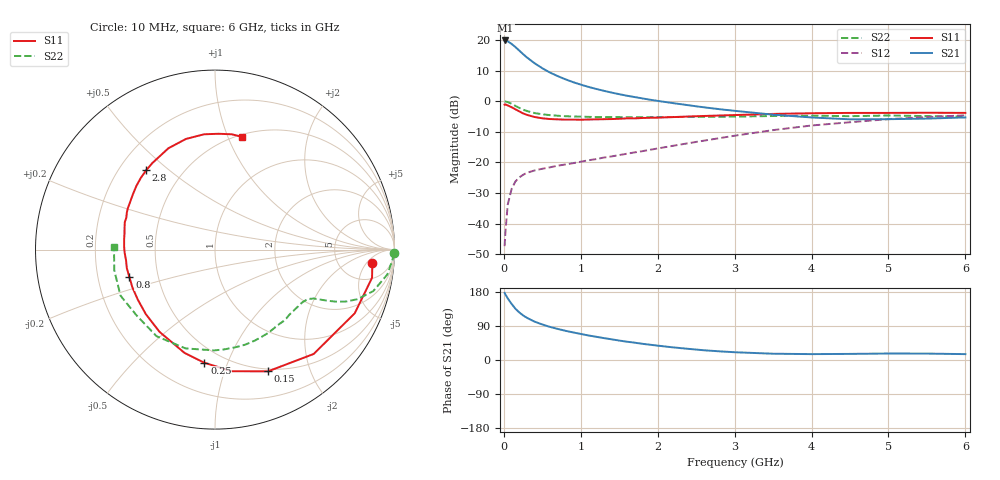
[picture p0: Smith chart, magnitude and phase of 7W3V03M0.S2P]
! Infineon Technologies  Discrete & RF Semiconductors
! BFS17W
! Si NPN RF Bipolar Junction Transistor in SOT323
! VCE = 3 V  IC = 3 mA
! Common Emitter S-Parameters:  August  1999
# GHz  S  MA  R  50
!  f  S11  S21  S12  S22
! GHz  MAG  ANG  MAG  ANG  MAG  ANG  MAG  ANG
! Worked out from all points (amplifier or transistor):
!   36 points, 10 MHz to 6 GHz, reference 50 ohm
!   highest |S21| = 19.9 dB at 20 MHz (marker M1)
!   |S21| within 3 dB of that: start of sweep to 187.2 MHz
!   unconditionally stable (mu >= 1): 699.9 MHz to 3.232 GHz; 4.015 GHz to end of sweep
!   at 250 MHz: K = 0.45, MSG = 19.7 dB, |S12| = -24.0 dB
!   at 1.4 GHz: K = 1.29, MAG = 7.2 dB, |S12| = -18.0 dB
!   at 6 GHz: K = 1.09, MAG = -2.2 dB, |S12| = -4.6 dB
!   S11 on the Smith chart (normalised r, x): 10 MHz: 11, -7; 150 MHz: 0.47, -1.42; 250 MHz: 0.39, -0.83; 800 MHz: 0.34, -0.14; 2.8 GHz: 0.31, +0.42; 6 GHz: 0.52, +1.12
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0.01  0.8798 -4.9  9.833 177.1  0.0043 85.5  0.9971 -1.2
0.02  0.889 -10.2  9.842 173.1  0.0071 85.8  0.9899 -3.4
0.05  0.8555 -24.5  9.54 162.9  0.0203 77.7  0.9704 -8.2
0.1  0.8003 -46.6  8.658 148.2  0.0367 65.7  0.9116 -14.7
0.15  0.7397 -66.5  7.69 135.4  0.0489 57.6  0.8405 -19.2
0.2  0.6843 -82.0  6.736 125.7  0.057 52.4  0.781 -21.8
0.25  0.6336 -95.3  5.896 117.7  0.0629 48.0  0.7293 -23.4
0.3  0.6002 -106.4  5.2 111.4  0.0678 45.8  0.6939 -24.3
0.4  0.5527 -124.0  4.176 101.2  0.0742 43.4  0.6419 -25.6
0.5  0.5271 -137.0  3.461 93.7  0.079 42.9  0.6125 -26.4
0.6  0.5125 -147.0  2.943 87.3  0.0834 43.8  0.5931 -27.6
0.8  0.5011 -162.1  2.285 77.1  0.0928 46.7  0.57 -30.8
0.9  0.502 -168.1  2.053 72.8  0.0975 48.2  0.5637 -32.6
1.1  0.5038 -178.1  1.717 64.7  0.1087 51.2  0.5562 -36.8
1.3  0.5097 173.3  1.483 57.8  0.1204 53.8  0.5505 -41.7
1.6  0.5253 163.1  1.232 48.3  0.139 57.6  0.5477 -49.3
2.2  0.5512 146.2  0.933 33.3  0.1875 62.6  0.5534 -66.4
2.8  0.5852 130.9  0.743 22.9  0.2494 62.9  0.5583 -84.7
3.5  0.6215 114.7  0.604 16.6  0.338 59.2  0.5745 -106.6
4.5  0.6454 95.4  0.507 16.1  0.4543 47.4  0.5704 -139.8
5.5  0.6493 81.7  0.521 16.9  0.5512 34.9  0.5728 -168.5
6  0.6458 76.6  0.545 15.5  0.5892 28.9  0.5628 178.8
